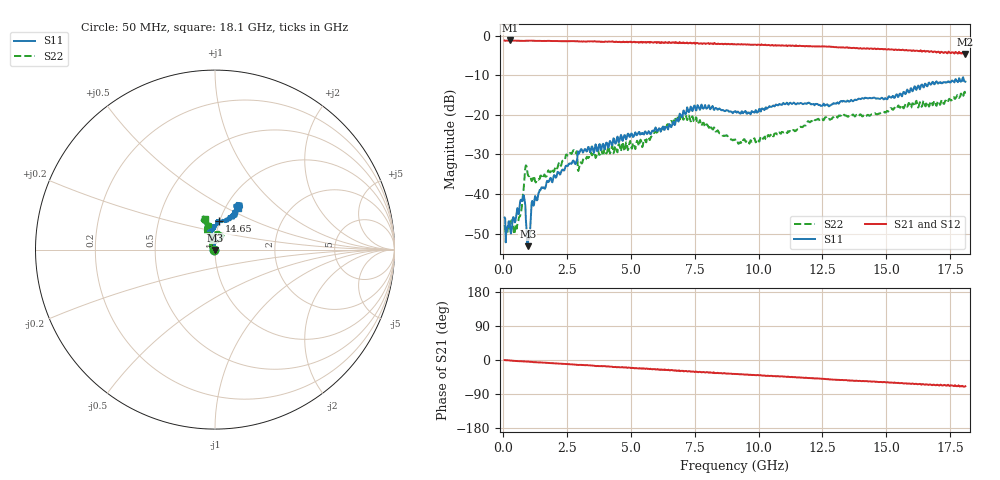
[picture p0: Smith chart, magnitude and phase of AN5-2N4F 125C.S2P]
! Network Analyzer HP8720D.06.14 Serial No. US36140669
! 12 Jan 2005  10:08:43
! Frequency  S11  S21  S12  S22
# HZ  S  DB R 50
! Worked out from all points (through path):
!   801 points, 50 MHz to 18.1 GHz, reference 50 ohm
!   highest |S21| = -1.23 dB at 253.1 MHz (marker M1); lowest = -4.7 dB at 18.1 GHz (marker M2)
!   group delay of S21, straight-line fit = 10.7 ps
!   lowest |S11| = -53.2 dB at 952.5 MHz (marker M3), VSWR 1.00, Z = 49.8 - j0.154 ohm
!   |S11| at or under -10 dB: start of sweep to end of sweep
!   |S22| runs from -50.2 to -14.2 dB; largest |S21 - S12| = 0.031
!   S11 on the Smith chart (normalised r, x): 50 MHz: 0.99, -0.01; 14.65 GHz: 0.99, +0.33; 18.1 GHz: 1.14, +0.56
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5e7  -45.94 -130.3  -1.26 -0.3  -1.30 -0.7  -47.93 -168.7
2.530625e8  -47.65 178.1  -1.23 -1.2  -1.25 -1.6  -48.67 -135.0
5.0125e8  -45.79 145.0  -1.29 -2.8  -1.28 -3.0  -47.87 -153.8
7.494375e8  -41.80 90.7  -1.33 -3.6  -1.32 -3.8  -41.56 -121.5
8.396875e8  -41.86 42.3  -1.32 -3.7  -1.33 -4.0  -35.39 -133.5
9.525e8  -53.20 -135.0  -1.31 -4.3  -1.28 -4.6  -34.93 172.9
1.020188e9  -51.20 154.6  -1.31 -4.5  -1.29 -4.9  -35.52 165.6
1.178125e9  -42.99 139.2  -1.30 -5.8  -1.33 -5.8  -35.46 156.5
1.471438e9  -38.68 124.0  -1.38 -6.6  -1.34 -6.9  -35.35 147.2
2.689812e9  -32.17 97.0  -1.39 -11.7  -1.39 -12.0  -29.72 129.9
2.802625e9  -32.36 90.7  -1.44 -12.2  -1.41 -12.7  -29.60 126.4
3.005688e9  -29.17 98.5  -1.49 -13.1  -1.47 -13.3  -32.53 161.8
3.073375e9  -28.79 93.0  -1.47 -13.2  -1.43 -13.4  -32.33 157.3
6.074188e9  -23.79 102.8  -1.72 -25.5  -1.73 -25.5  -24.22 107.5
7.066938e9  -18.92 97.5  -1.78 -30.0  -1.81 -29.4  -21.21 78.0
7.834062e9  -18.45 93.5  -1.98 -31.7  -1.92 -32.6  -22.02 61.7
9.075e9  -19.17 106.7  -2.20 -36.7  -2.15 -37.1  -26.27 70.7
9.954938e9  -19.41 106.8  -2.31 -39.5  -2.29 -40.4  -26.19 83.9
1.209838e10  -17.33 100.0  -2.71 -48.1  -2.68 -48.4  -21.66 102.8
1.464794e10  -15.84 82.1  -3.33 -57.6  -3.33 -57.6  -19.90 117.4
1.509919e10  -15.33 75.9  -3.45 -59.4  -3.43 -59.5  -18.85 118.6
1.81e10  -11.63 61.3  -4.66 -69.3  -4.64 -71.9  -14.97 107.4
